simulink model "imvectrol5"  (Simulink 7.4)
settings: Solver=ode23tb  StartTime=0.0  StopTime=1  RelTol=1e-3  AbsTol=1e-3
InitFcn:
  | load('IC3.mat')

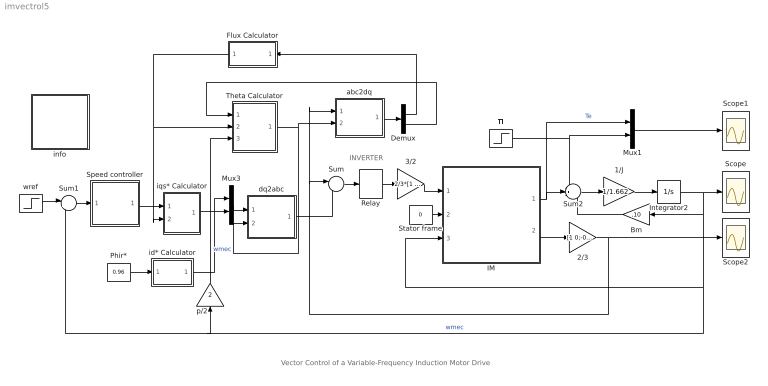
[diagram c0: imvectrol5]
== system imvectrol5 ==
  note: Vector Control of a Variable-Frequency Induction Motor Drive
  note: INVERTER
  1/J : Gain  Gain=1/1.662  ParameterDataType=sfix(16)  ParameterScaling=2^0  OutDataType=sfix(16)  OutScaling=2^0
  2/3 : Gain  Gain=[1 0;-0.5 sqrt(3)/2;-0.5 -sqrt(3)/2]  Multiplication=Matrix(K*u)  ParameterDataType=sfix(16)  ParameterScaling=2^0  OutDataType=sfix(16)  OutScaling=2^0
  3/2 : Gain  Gain=2/3*[1 -.5 -.5;0 sqrt(3)/2 -sqrt(3)/2]  Multiplication=Matrix(K*u)  ParameterDataType=sfix(16)  ParameterScaling=2^0  OutDataType=sfix(16)  OutScaling=2^0
  Bm : Gain  Gain=.10  ParameterDataType=sfix(16)  ParameterScaling=2^0  OutDataType=sfix(16)  OutScaling=2^0
  Demux : Demux  Outputs=2
  Flux Calculator : Subsystem
  IM : Subsystem  mask{Rs=0.087, Lsl=0.8e-3, Rr=0.228, Lrl=0.8e-3, Lm=34.7e-3, p=4}
      mask prompts: Rs "Stator resistance [ohm]"; Lsl "Stator leakage inductance [H]"; Rr "Rotor resistance [ohm]"; Lrl "Rotor leakage inductance [H]"; Lm "Magnetizing inductance [H]"; p "Number of poles"
  Integrator2 : Integrator
  Mux1 : Mux  Inputs=2
  Mux3 : Mux  Inputs=2
  Phir* : Constant  Value=0.96  OutDataType=sfix(16)  OutScaling=2^0
  Relay : Relay  OnSwitchValue=10  OffSwitchValue=-10  OnOutputValue=780  OffOutputValue=-780  OutDataType=sfix(16)  OutScaling=2^0
  Scope : Scope
  Scope1 : Scope
  Scope2 : Scope
  Speed controller : Subsystem  mask(PI controller){Kp=100, Ki=5200, Tlim=300, Ts=0}
      mask prompts: Kp "Proportional gain (Kp)"; Ki "Integral gain (Ki)"; Tlim "Torque limit (N.m)"; Ts "Sampling time (s)"
      mask help: Proportional-Integral Speed Controller
  Stator frame : Constant  Value=0  OutDataType=sfix(16)  OutScaling=2^0
  Sum : Sum  Inputs=|-+  OutDataType=sfix(16)  OutScaling=2^0
  Sum1 : Sum  Inputs=|+-  OutDataType=sfix(16)  OutScaling=2^0
  Sum2 : Sum  Inputs=-+-  OutDataType=sfix(16)  OutScaling=2^0
  Theta Calculator : Subsystem
  Tl : Step  Time=0.6  After=200  SampleTime=0
  abc2dq : Subsystem
  dq2abc : Subsystem
  id* Calculator : Subsystem
  info : Subsystem
  iqs* Calculator : Subsystem
  p/2 : Gain  Gain=2  ParameterDataType=sfix(16)  ParameterScaling=2^0  OutDataType=sfix(16)  OutScaling=2^0
  wref : Step  Time=0.1  Before=120  After=150  SampleTime=0
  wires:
  Phir*/1 -> id* Calculator/1(Phir*)
  iqs* Calculator/1(Iq*) -> Mux3/2
  id* Calculator/1(Id*) -> Mux3/1
  Flux Calculator/1(Phir) -> Theta Calculator/2(Phir), iqs* Calculator/2(Phir)
  wref/1 -> Sum1/1
  Sum2/1 -> 1/J/1
  1/J/1 -> Integrator2/1
  Integrator2/1 -> Bm/1, IM/3(wmec), Sum1/2, p/2/1, Scope/1  "wmec"
  Bm/1 -> Sum2/3
  IM/1(Te) -> Sum2/2, Mux1/1  "Te"
  Stator frame/1 -> IM/2(wk)
  IM/2(is) -> 2/3/1
  2/3/1 -> Scope2/1, Sum/1, abc2dq/1(iabc)
  Sum/1 -> Relay/1
  3/2/1 -> IM/1(vs)
  Relay/1 -> 3/2/1
  Mux3/1 -> dq2abc/1(idq)
  dq2abc/1(iabc^) -> Sum/2
  Theta Calculator/1(theta) -> dq2abc/2(theta), abc2dq/2(theta)
  Demux/1 -> Flux Calculator/1(Id)
  Demux/2 -> Theta Calculator/1(Iq)
  Speed controller/1(Te*) -> iqs* Calculator/1(Te*)
  Sum1/1 -> Speed controller/1(we)
  abc2dq/1(idq) -> Demux/1
  p/2/1 -> Theta Calculator/3(wm)  "wmec"
  Mux1/1 -> Scope1/1
  Tl/1 -> Mux1/2, Sum2/1  "Tl"

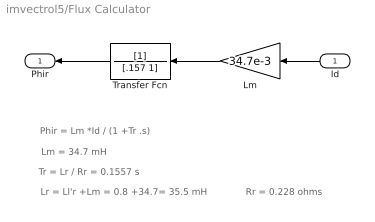
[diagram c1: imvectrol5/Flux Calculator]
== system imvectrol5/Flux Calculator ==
  note: Phir = Lm *Id / (1 +Tr .s)
  note: Lm = 34.7 mH
  note: Lr = Ll'r +Lm = 0.8 +34.7= 35.5 mH
  note: Tr = Lr / Rr = 0.1557 s
  note: Rr = 0.228 ohms
  Id : Inport  OutDataType=sfix(16)  OutScaling=2^0
  Lm : Gain  Gain=34.7e-3  ParameterDataType=sfix(16)  ParameterScaling=2^0  OutDataType=sfix(16)  OutScaling=2^0
  Transfer Fcn : TransferFcn  Denominator=[.157 1]
  Phir : Outport
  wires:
  Transfer Fcn/1 -> Phir/1
  Id/1 -> Lm/1
  Lm/1 -> Transfer Fcn/1

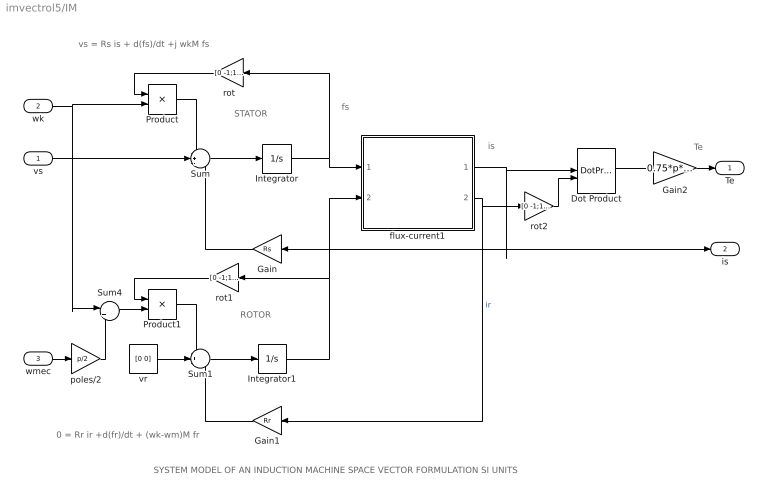
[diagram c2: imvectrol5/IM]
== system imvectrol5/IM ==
  note: 0 = Rr ir +d(fr)/dt + (wk-wm)M fr
  note: vs = Rs is + d(fs)/dt +j wkM fs
  note: SYSTEM MODEL OF AN INDUCTION MACHINE SPACE VECTOR FORMULATION SI UNITS
  note: Te
  note: is
  note: fs
  note: STATOR
  note: ROTOR
  vs : Inport  OutDataType=sfix(16)  OutScaling=2^0
  wk : Inport  Port=2  OutDataType=sfix(16)  OutScaling=2^0
  wmec : Inport  Port=3  OutDataType=sfix(16)  OutScaling=2^0
  Dot Product : DotProduct  OutDataType=fixdt(1, 16)  OutScaling=2^-10
  Gain : Gain  Gain=Rs  ParameterDataType=sfix(16)  ParameterScaling=2^0  OutDataType=sfix(16)  OutScaling=2^0
  Gain1 : Gain  Gain=Rr  ParameterDataType=sfix(16)  ParameterScaling=2^0  OutDataType=sfix(16)  OutScaling=2^0
  Gain2 : Gain  Gain=0.75*p*Lm  ParameterDataType=sfix(16)  ParameterScaling=2^0  OutDataType=sfix(16)  OutScaling=2^0
  Integrator : Integrator  InitialCondition=[0 0]
  Integrator1 : Integrator  InitialCondition=[0 0]
  Product : Product  OutDataType=sfix(16)  OutScaling=2^0
  Product1 : Product  OutDataType=sfix(16)  OutScaling=2^0
  Sum : Sum  Inputs=-+-  OutDataType=sfix(16)  OutScaling=2^0
  Sum1 : Sum  Inputs=-+-  OutDataType=sfix(16)  OutScaling=2^0
  Sum4 : Sum  Inputs=|+-  OutDataType=sfix(16)  OutScaling=2^0
  flux-current1 : Subsystem
  poles/2 : Gain  Gain=p/2  ParameterDataType=sfix(16)  ParameterScaling=2^0  OutDataType=sfix(16)  OutScaling=2^0
  rot : Gain  Gain=[0 -1;1 0]  Multiplication=Matrix(K*u)  ParameterDataType=sfix(16)  ParameterScaling=2^0  OutDataType=sfix(16)  OutScaling=2^0
  rot1 : Gain  Gain=[0 -1;1 0]  Multiplication=Matrix(K*u)  ParameterDataType=sfix(16)  ParameterScaling=2^0  OutDataType=sfix(16)  OutScaling=2^0
  rot2 : Gain  Gain=[0 -1;1 0]  Multiplication=Matrix(K*u)  ParameterDataType=sfix(16)  ParameterScaling=2^0  OutDataType=sfix(16)  OutScaling=2^0
  vr : Constant  Value=[0 0]  OutDataType=sfix(16)  OutScaling=2^0
  Te : Outport
  is : Outport  Port=2
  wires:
  poles/2/1 -> Sum4/2
  wmec/1 -> poles/2/1
  Gain2/1 -> Te/1
  Dot Product/1 -> Gain2/1
  flux-current1/2(ir) -> rot2/1, Gain1/1  "ir"
  flux-current1/1(is) -> is/1, Gain/1, Dot Product/1
  Sum/1 -> Integrator/1
  Sum1/1 -> Integrator1/1
  wk/1 -> Sum4/1, Product/2
  vs/1 -> Sum/2
  Sum4/1 -> Product1/2
  rot/1 -> Product/1
  Product/1 -> Sum/1
  rot1/1 -> Product1/1
  Product1/1 -> Sum1/1
  Integrator1/1 -> rot1/1, flux-current1/2(fr)
  Integrator/1 -> rot/1, flux-current1/1(fs)
  Gain1/1 -> Sum1/3
  vr/1 -> Sum1/2
  Gain/1 -> Sum/3
  rot2/1 -> Dot Product/2

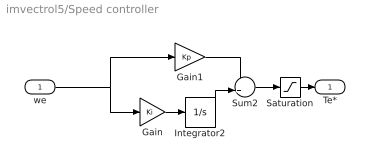
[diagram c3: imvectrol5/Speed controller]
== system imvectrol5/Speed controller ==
  we : Inport  OutDataType=sfix(16)  OutScaling=2^0
  Gain : Gain  Gain=Ki  ParameterDataType=sfix(16)  ParameterScaling=2^0  OutDataType=sfix(16)  OutScaling=2^0
  Gain1 : Gain  Gain=Kp  ParameterDataType=sfix(16)  ParameterScaling=2^0  OutDataType=sfix(16)  OutScaling=2^0
  Integrator2 : Integrator  LimitOutput=on  UpperSaturationLimit=Tlim  LowerSaturationLimit=-Tlim
  Saturation : Saturate  UpperLimit=Tlim  LowerLimit=-Tlim
  Sum2 : Sum  OutDataType=sfix(16)  OutScaling=2^0
  Te* : Outport  InitialOutput=0
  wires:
  Gain1/1 -> Sum2/1
  Gain/1 -> Integrator2/1
  Saturation/1 -> Te*/1
  we/1 -> Gain/1, Gain1/1
  Sum2/1 -> Saturation/1
  Integrator2/1 -> Sum2/2

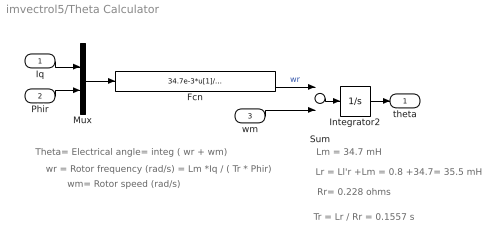
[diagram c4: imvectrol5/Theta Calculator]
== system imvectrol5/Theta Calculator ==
  note: Theta= Electrical angle= integ ( wr + wm)
  note: wr = Rotor frequency (rad/s) = Lm *Iq / ( Tr * Phir)
  note: Lm = 34.7 mH
  note: Rr= 0.228 ohms
  note: Lr = Ll'r +Lm = 0.8 +34.7= 35.5 mH
  note: wm= Rotor speed (rad/s)
  note: Tr = Lr / Rr = 0.1557 s
  Iq : Inport  OutDataType=sfix(16)  OutScaling=2^0
  Phir : Inport  Port=2  OutDataType=sfix(16)  OutScaling=2^0
  wm : Inport  Port=3  OutDataType=sfix(16)  OutScaling=2^0
  Fcn : Fcn  Expr=34.7e-3*u[1]/(u[2]*0.1557+1e-3)
  Integrator2 : Integrator
  Mux : Mux  Inputs=2
  Sum : Sum  OutDataType=sfix(16)  OutScaling=2^0
  theta : Outport  InitialOutput=0
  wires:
  Integrator2/1 -> theta/1
  Sum/1 -> Integrator2/1
  wm/1 -> Sum/2
  Fcn/1 -> Sum/1  "wr"
  Phir/1 -> Mux/2
  Iq/1 -> Mux/1
  Mux/1 -> Fcn/1

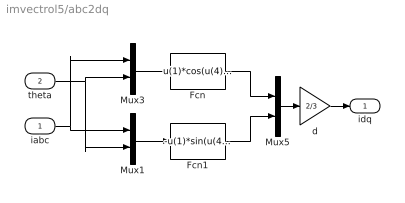
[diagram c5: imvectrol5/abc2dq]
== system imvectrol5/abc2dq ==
  iabc : Inport  OutDataType=sfix(16)  OutScaling=2^0
  theta : Inport  Port=2  OutDataType=sfix(16)  OutScaling=2^0
  Fcn : Fcn  Expr=u(1)*cos(u(4))+u(2)*cos(u(4)-2*pi/3)+u(3)*cos(u(4)+2*pi/3)
  Fcn1 : Fcn  Expr=-u(1)*sin(u(4))-u(2)*sin(u(4)-2*pi/3)-u(3)*sin(u(4)+2*pi/3)
  Mux1 : Mux  Inputs=2
  Mux3 : Mux  Inputs=2
  Mux5 : Mux  Inputs=2
  d : Gain  Gain=2/3  ParameterDataType=sfix(16)  ParameterScaling=2^0  OutDataType=sfix(16)  OutScaling=2^0
  idq : Outport
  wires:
  Mux3/1 -> Fcn/1
  Fcn/1 -> Mux5/1
  Mux5/1 -> d/1
  Mux1/1 -> Fcn1/1
  Fcn1/1 -> Mux5/2
  iabc/1 -> Mux1/1, Mux3/1
  theta/1 -> Mux3/2, Mux1/2
  d/1 -> idq/1

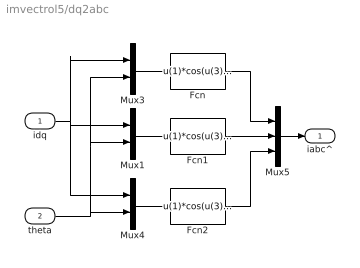
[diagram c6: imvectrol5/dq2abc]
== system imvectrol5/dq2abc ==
  idq : Inport  OutDataType=sfix(16)  OutScaling=2^0
  theta : Inport  Port=2  OutDataType=sfix(16)  OutScaling=2^0
  Fcn : Fcn  Expr=u(1)*cos(u(3))-u(2)*sin(u(3))
  Fcn1 : Fcn  Expr=u(1)*cos(u(3)-2*pi/3)-u(2)*sin(u(3)-2*pi/3)
  Fcn2 : Fcn  Expr=u(1)*cos(u(3)+2*pi/3)-u(2)*sin(u(3)+2*pi/3)
  Mux1 : Mux  Inputs=2
  Mux3 : Mux  Inputs=2
  Mux4 : Mux  Inputs=2
  Mux5 : Mux  Inputs=3
  iabc^ : Outport
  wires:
  Mux3/1 -> Fcn/1
  Mux4/1 -> Fcn2/1
  idq/1 -> Mux3/1, Mux4/1, Mux1/1
  Fcn/1 -> Mux5/1
  Mux5/1 -> iabc^/1
  Mux1/1 -> Fcn1/1
  Fcn1/1 -> Mux5/2
  Fcn2/1 -> Mux5/3
  theta/1 -> Mux4/2, Mux3/2, Mux1/2

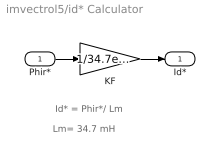
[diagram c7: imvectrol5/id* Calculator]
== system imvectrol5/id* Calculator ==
  note: Id* = Phir*/ Lm
  note: Lm= 34.7 mH
  Phir* : Inport  OutDataType=sfix(16)  OutScaling=2^0
  KF : Gain  Gain=1/34.7e-3  ParameterDataType=sfix(16)  ParameterScaling=2^0  OutDataType=sfix(16)  OutScaling=2^0
  Id* : Outport
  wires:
  KF/1 -> Id*/1
  Phir*/1 -> KF/1

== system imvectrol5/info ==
  note: A three-phase induction motor rated at 50hp, 460V,4pole,60Hz is modeled in the common stator reference frame.The speed loop utilizes a PI controller to produce the quadrature-axis currents iq* which serves as the torque command. The derived direct-axis current id* serves as the rotor flux command. These currents are then transformed via the block into the currrent references ia*, ib*, and ic* fed into the current regulator. The current-controlled PWM inverter is made up of three hysteresis controllers. Rotor flux field orientation is obtained in the block. The machine is initially operating in steady state at no load (Tl=0) at the speed wref=120rad/s. Examine the transient response due to step changes in the command speed wref and load torque Tl. Repeat the simulation for a so-called detuned case when the estimated value of the rotor time constant Tr appearing in the differs from the actual value used for the motor parameters.
  note: (adapted from Power System Blockset case study)
  note: Indirect Vector Control of a Variable-Frequency Induction Motor Drive

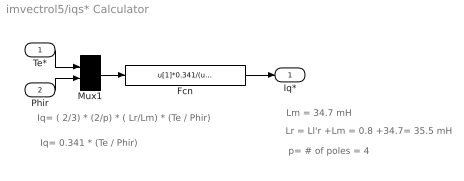
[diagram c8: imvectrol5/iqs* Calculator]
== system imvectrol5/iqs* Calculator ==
  note: Iq= ( 2/3) * (2/p) * ( Lr/Lm) * (Te / Phir)
  note: Lm = 34.7 mH
  note: Lr = Ll'r +Lm = 0.8 +34.7= 35.5 mH
  note: p= # of poles = 4
  note: Iq= 0.341 * (Te / Phir)
  Te* : Inport  OutDataType=sfix(16)  OutScaling=2^0
  Phir : Inport  Port=2  OutDataType=sfix(16)  OutScaling=2^0
  Fcn : Fcn  Expr=u[1]*0.341/(u[2]+1e-3)
  Mux1 : Mux  Inputs=2
  Iq* : Outport  InitialOutput=0
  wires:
  Phir/1 -> Mux1/2
  Fcn/1 -> Iq*/1
  Te*/1 -> Mux1/1
  Mux1/1 -> Fcn/1

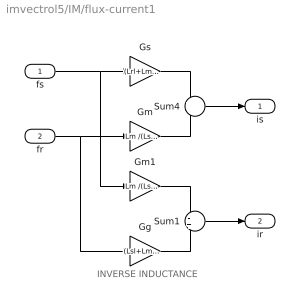
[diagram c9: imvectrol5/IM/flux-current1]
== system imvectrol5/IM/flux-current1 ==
  note: INVERSE INDUCTANCE
  fs : Inport  OutDataType=sfix(16)  OutScaling=2^0
  fr : Inport  Port=2  OutDataType=sfix(16)  OutScaling=2^0
  Gg : Gain  Gain=(Lsl+Lm )/(Lsl*Lrl+Lsl*Lm+Lrl*Lm)  ParameterDataType=sfix(16)  ParameterScaling=2^0  OutDataType=sfix(16)  OutScaling=2^0
  Gm : Gain  Gain=Lm /(Lsl*Lrl+Lsl*Lm+Lrl*Lm)  ParameterDataType=sfix(16)  ParameterScaling=2^0  OutDataType=sfix(16)  OutScaling=2^0
  Gm1 : Gain  Gain=Lm /(Lsl*Lrl+Lsl*Lm+Lrl*Lm)  ParameterDataType=sfix(16)  ParameterScaling=2^0  OutDataType=sfix(16)  OutScaling=2^0
  Gs : Gain  Gain=(Lrl+Lm) /(Lsl*Lrl+Lsl*Lm+Lrl*Lm)  ParameterDataType=sfix(16)  ParameterScaling=2^0  OutDataType=sfix(16)  OutScaling=2^0
  Sum1 : Sum  Inputs=-+  OutDataType=sfix(16)  OutScaling=2^0
  Sum4 : Sum  Inputs=+-  OutDataType=sfix(16)  OutScaling=2^0
  is : Outport
  ir : Outport  Port=2
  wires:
  fs/1 -> Gs/1, Gm1/1
  Gs/1 -> Sum4/1
  fr/1 -> Gm/1, Gg/1
  Gm/1 -> Sum4/2
  Sum4/1 -> is/1
  Gm1/1 -> Sum1/1
  Gg/1 -> Sum1/2
  Sum1/1 -> ir/1
